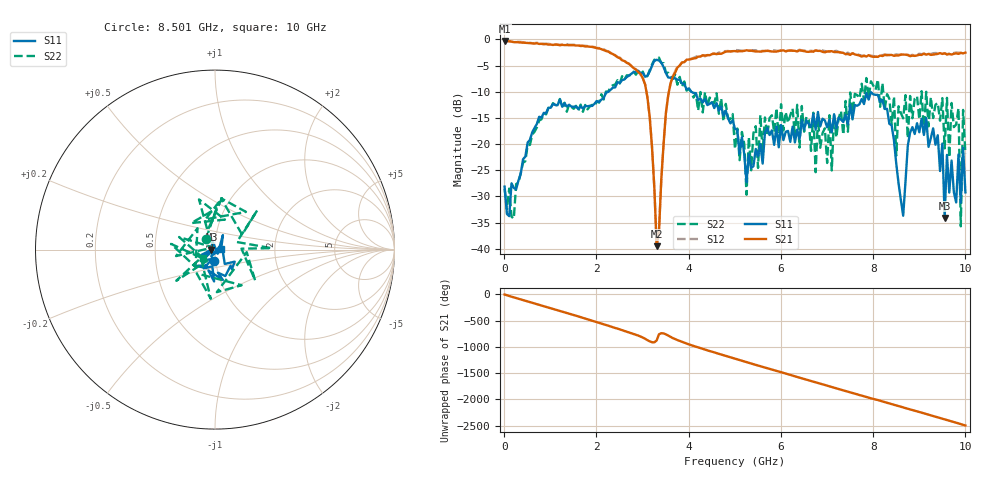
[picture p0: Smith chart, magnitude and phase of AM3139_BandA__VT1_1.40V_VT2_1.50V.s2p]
! Date/Time: Tue, Nov 13, 2018 4:57 PM
! Network Analyzer: Agilent Technologies E8364B Rev: A.07.50.67
! Sweep from 0.010 to 10.000 GHz, 201 Points, Sweep Type: LIN
! Power Supply: 1.400 V, 0.000 A
# Hz S DB R 50
!freq MagS11 AngS11 MagS21 AngS21 MagS12 AngS12 MagS22 AngS22
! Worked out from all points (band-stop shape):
!   201 points, 10 MHz to 10 GHz, reference 50 ohm
!   highest |S21| = -0.31 dB at 10 MHz (marker M1); lowest = -39.5 dB at 3.307 GHz (marker M2)
!   |S21| within 3 dB of the highest: start of sweep to 2.445 GHz; 4.2 GHz to 7.994 GHz (3.793 GHz wide, 62.2 % of centre)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
!   lowest |S11| = -34.1 dB at 9.55 GHz (marker M3), VSWR 1.04, Z = 48.1 - j0.0348 ohm
!   |S11| at or under -10 dB: start of sweep to 2.259 GHz; 4.059 GHz to end of sweep
!   |S22| runs from -35.7 to -3.5 dB; largest |S21 - S12| = 0.028
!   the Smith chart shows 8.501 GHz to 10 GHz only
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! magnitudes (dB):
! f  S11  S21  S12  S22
! 10 MHz  -28.1  -0.3  -0.2  -28.6
! 1.708 GHz  -13.2  -1.2  -1.2  -13.8
! 3.057 GHz  -7.1  -8.6  -8.6  -7.3
! 3.307 GHz  -3.9  -39.5  -39.3  -4.1
! 3.357 GHz  -4.0  -36.8  -36.4  -3.5
! 3.656 GHz  -7.5  -7.1  -7.1  -7.5
! 5.005 GHz  -17.1  -2.2  -2.0  -21.0
! 5.255 GHz  -27.3  -2.1  -2.2  -29.7
! 5.554 GHz  -20.0  -2.3  -2.2  -14.4
! 6.703 GHz  -14.2  -2.3  -2.2  -14.0
! 7.103 GHz  -17.8  -2.2  -2.2  -25.0
! 7.502 GHz  -12.4  -2.9  -2.8  -10.1
! 8.352 GHz  -16.1  -3.0  -3.0  -11.3
! 8.651 GHz  -33.7  -2.9  -2.8  -15.1
! 8.851 GHz  -16.8  -3.1  -2.9  -15.1
! 9.401 GHz  -18.3  -2.8  -2.6  -12.1
! 9.55 GHz  -34.1  -2.6  -2.6  -20.8
! 9.6 GHz  -22.1  -2.9  -2.8  -11.2
! 9.85 GHz  -22.0  -2.8  -2.5  -13.1
! 9.9 GHz  -31.2  -2.6  -2.5  -35.7
! 9.95 GHz  -20.7  -2.7  -2.7  -13.5
! 10 GHz  -29.2  -2.5  -2.4  -21.9
